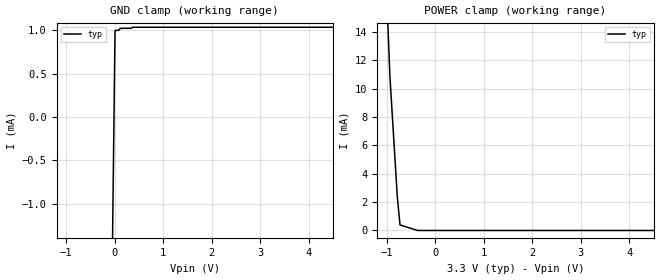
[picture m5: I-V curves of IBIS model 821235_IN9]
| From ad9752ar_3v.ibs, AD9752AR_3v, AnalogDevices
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| COPYRIGHT(C) MENTOR GRAPHICS CORPORATION 2002 ALL
| RIGHTS RESERVED. THIS WORK CONTAINS PROPRIETARY
| INFORMATION WHICH IS THE PROPERTY OF MENTOR GRAPHICS
| CORPORATION OR ITS LICENSORS. USE OF THESE MATERIALS
| IS SUBJECT TO THE TERMS BELOW.
| USE: MENTOR GRAPHICS HAS LICENSED IBIS MODELS TO
| SPECIFIC INTEGRATED CIRCUIT SUPPLIERS ("IC VENDORS")
| FOR USE AND DISTRIBUTION AS FOLLOWS: EACH IC VENDOR
| MAY USE IBIS MODELS, AND DISTRIBUTE THEM TO IC VENDOR'S
| CUSTOMERS TO USE, SOLELY FOR DEVELOPING PRINTED
| CIRCUIT BOARD DESIGNS. NO OTHER USE OR DISTRIBUTION
| OF THESE MATERIALS IS PERMITTED.
| Model Application Version 1.89 2/18/99.
[Model] 821235_IN9
Model_type Input
Vinl = 900.0mV
Vinh = 2.100V
C_comp 5.000pF NA NA
| variable typ   min   max
[Voltage Range] 3.300V NA NA
[GND Clamp Reference] 0.000V NA NA
[POWER Clamp Reference] 3.300V NA NA
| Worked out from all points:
|   POWER clamp passes 1 mA (typ) near -0.75 V on its own axis
[GND Clamp]
-3.3V     -155.8mA   NA         NA
5.334mV   998.3uA    NA         NA
35.71mV   998.3uA    NA         NA
66.08mV   1.003mA    NA         NA
88.85mV   1.003mA    NA         NA
111.6mV   1.024mA    NA         NA
339.7mV   1.024mA    NA         NA
365.1mV   1.036mA    NA         NA
6.6V      1.036mA    NA         NA
[POWER Clamp]
-3.3V     262.9mA    NA         NA
-1.104V   25.22mA    NA         NA
-936.8mV  10.84mA    NA         NA
-784.8mV  2.382mA    NA         NA
-728.9mV  390.4uA    NA         NA
-364.5mV  0A         NA         NA
6.6V      0A         NA         NA
